{attribute 'qualified_only'}
TYPE E_FunctionType :
(
	Sine,		// typical for vibrations originating from rotating machine
	Square,		// mixed sine signals good for analyzing spectrum
	Pulse,		// mixed sine signals good for analyzing spectrum
	Triangular,	// mixed sine signals good for analyzing spectrum
	Sawtooth,	// ramp-type vibrations, continuously increasing
	AM			// amplitude modulation: typical for vibrations originating from gear-tooth failure or bearing faults
);
END_TYPE
